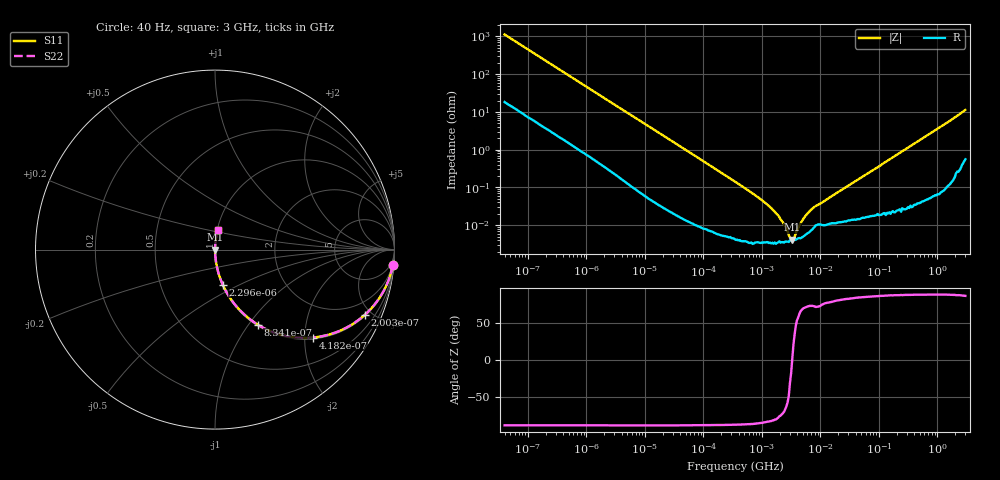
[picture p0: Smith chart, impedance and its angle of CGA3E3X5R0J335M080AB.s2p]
! S-parameter Generated by TDK Corporation
! Copyright(C) 2015 TDK Corporation.
! All Rights Reserved.
! TDK P/N: CGA3E3X5R0J335M080AB (Multilayer Ceramic Chip Capacitors)
! Property: C=3.3uF
! Size(LxWxT): 1.6x0.8x0.8mm, 0.063x0.031x0.031inches
! Model Type: s2p (Touchstone File Format Version 1.0)
! Frequency: DC=Yes Start=0.00004MHz Stop=3000MHz 396points Log-sweep
! Note: This model was converted from impedance.
! Model Generated on Jun. 23, 2015
! Hash(MD5):
! Port Assignments:
!  1 ---| |--- 2
! Applicable Conditions:
!  Temperature = 25 degC
!  DC Bias Voltage = 0 V
!  Small Signal Operation
! Terms and conditions regarding TDK Simulation Models
! (1)This simulation model is being provided solely for informational purposes. Please refer to the specifications of the products in terms of detailed characteristics of such products.
! (2)In no event shall TDK Corporation of any of its subsidiaries be liable for any loss or damage arising, directly or indirectly,
!  From any information contained in this simulation model, including, but not limited to loss or damages arising from any inaccuracies, omissions or errors in connection with such information.
! (3)Any and all copyrights on this simulation model are owned by TDK Corporation.
!  Duplication or redistribution of this simulation model without prior written permission from TDK Corporation is prohibited.
! (4)This simulation model is subject to any modification or change without any prior notice.
! (5)Neither TDK Corporation nor any of its subsidiaries shall make any warranty, express or implied,
!  Including but not limited to the correctness, implied warranties of merchantability and fitness for a particular purpose with respect to this simulation models.
! (6)The use of this simulation model shall be deemed to have consented to the terms and conditions hereof.
# MHz S MA R 50
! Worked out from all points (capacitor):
!   395 points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, 40 Hz to 3 GHz, reference 50 ohm
!   read as one part in series: C = 3.52 uF near 41.88 Hz
!   lowest |Z| = 4.11 mohm at 3.304 MHz (marker M1)
!   series resonance near 3.285 MHz, so ESL is about 670 pH
!   S11 on the Smith chart (normalised r, x): 40 Hz: 1, -23; 200.3 Hz: 1.07, -4.56; 418.2 Hz: 1.04, -2.20; 834.1 Hz: 1.02, -1.11; 2.296 kHz: 1.01, -0.41; 3 GHz: 1.01, +0.23
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4e-05  0.9947 -5.0  0.088 84.0  0.088 84.0  0.9947 -5.0
0.000105147  0.9709 -13.0  0.2245 76.1  0.2245 76.1  0.9709 -13.0
0.0002002725  0.9106 -23.5  0.399 65.6  0.399 65.6  0.9106 -23.5
0.000289415  0.8394 -32.0  0.5301 57.1  0.5301 57.1  0.8394 -32.0
0.0004182353  0.7338 -41.9  0.6676 47.2  0.6676 47.2  0.7338 -41.9
0.0005772088  0.6192 -50.8  0.7754 38.2  0.7754 38.2  0.6192 -50.8
0.000834128  0.4818 -60.3  0.8687 28.8  0.8687 28.8  0.4818 -60.3
0.001321622  0.3306 -69.8  0.9386 19.3  0.9386 19.3  0.3306 -69.8
0.002295921  0.1998 -77.6  0.9768 11.5  0.9768 11.5  0.1998 -77.6
0.005504511  0.08641 -84.3  0.9951 5.0  0.9951 5.0  0.08641 -84.3
0.01739424  0.02797 -87.7  0.9993 1.6  0.9993 1.6  0.02797 -87.7
0.3464102  0.001428 -88.2  1 0.1  1 0.1  0.001428 -88.2
1.146211  0.0003887 -84.9  1 0.0  1 0.0  0.0003887 -84.9
1.816098  0.000195 -79.9  1 0.0  1 0.0  0.000195 -79.9
2.393669  0.0001044 -70.5  1 0.0  1 0.0  0.0001044 -70.5
3.303516  4.11e-05 2.5  1 -0.0  1 -0.0  4.11e-05 2.5
4.354128  9.824e-05 62.3  1 -0.0  1 -0.0  9.824e-05 62.3
5.480732  0.0001722 71.4  0.9999 -0.0  0.9999 -0.0  0.0001722 71.4
7.22376  0.0002722 73.7  0.9999 -0.0  0.9999 -0.0  0.0002722 73.7
150.6385  0.0055 87.4  0.9998 -0.3  0.9998 -0.3  0.0055 87.4
994.0817  0.03533 86.9  0.9987 -2.0  0.9987 -2.0  0.03533 86.9
3000  0.1122 80.7  0.9882 -6.4  0.9882 -6.4  0.1122 80.7
